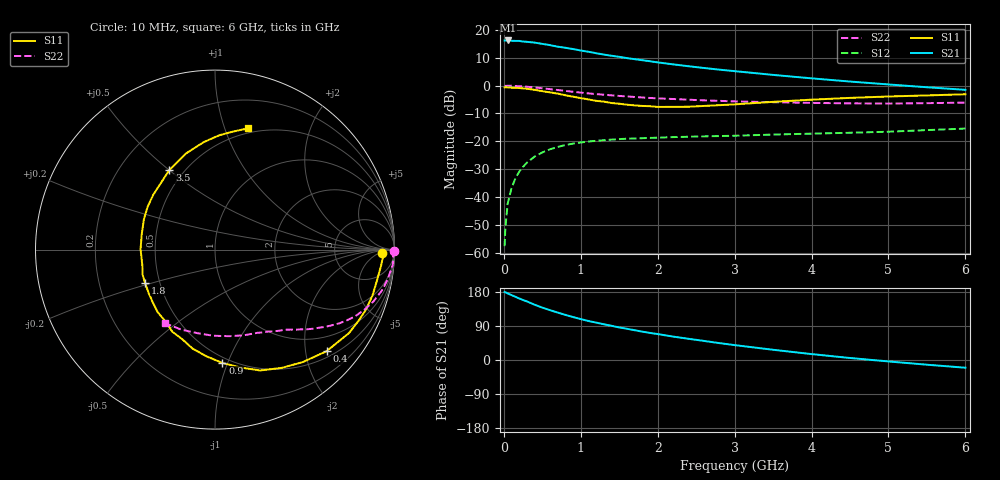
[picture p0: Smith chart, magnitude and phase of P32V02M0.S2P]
! SIEMENS Small Signal Semiconductors
! BFP181
! Si NPN RF Bipolar Junction Transistor in SOT143
! VCE = 2 V  IC = 2 mA
! Common Emitter S-Parameters:  March  1996
# GHz  S  MA  R  50
!  f  S11  S21  S12  S22
! GHz  MAG  ANG  MAG  ANG  MAG  ANG  MAG  ANG
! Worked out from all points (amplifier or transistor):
!   36 points, 10 MHz to 6 GHz, reference 50 ohm
!   highest |S21| = 16.2 dB at 50 MHz (marker M1)
!   |S21| within 3 dB of that: start of sweep to 881 MHz
!   unconditionally stable (mu >= 1): 2.395 GHz to end of sweep
!   at 250 MHz: K = 0.13, MSG = 22.5 dB, |S12| = -29.2 dB
!   at 1.4 GHz: K = 0.66, MSG = 15.1 dB, |S12| = -19.4 dB
!   at 6 GHz: K = 1.15, MAG = 4.6 dB, |S12| = -15.4 dB
!   lowest NFmin = 1.35 dB at 450 MHz
!   S11 on the Smith chart (normalised r, x): 10 MHz: 25, -8; 400 MHz: 0.63, -2.44; 900 MHz: 0.45, -0.96; 1.8 GHz: 0.41, -0.19; 3.5 GHz: 0.42, +0.50; 6 GHz: 0.45, +1.20
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0.01  0.9302 -1.3  6.469 179.4  0.0013 80.8  0.9969 -0.4
0.02  0.9375 -2.1  6.471 178.8  0.0028 89.9  0.9896 -0.9
0.05  0.9298 -5.5  6.487 175.6  0.0076 88.5  0.9938 -2.5
0.1  0.9185 -10.9  6.404 171.3  0.0144 82.8  0.9939 -4.9
0.2  0.905 -21.8  6.361 162.4  0.0284 76.6  0.9768 -9.6
0.3  0.8797 -31.9  6.126 154.6  0.0411 71.0  0.9553 -14.1
0.4  0.8408 -42.3  5.937 145.8  0.0531 65.2  0.9283 -18.2
0.5  0.7952 -52.0  5.629 138.2  0.0629 59.5  0.8962 -22.0
0.6  0.7561 -60.7  5.346 131.5  0.0717 54.7  0.8653 -25.4
0.7  0.719 -69.5  5.017 125.1  0.079 50.8  0.8337 -28.2
0.8  0.671 -78.0  4.796 119.0  0.0856 46.9  0.8049 -30.7
0.9  0.6326 -86.3  4.546 113.3  0.0908 43.5  0.775 -33.0
1.1  0.5653 -102.8  4.067 102.9  0.0988 37.9  0.725 -36.9
1.3  0.5156 -117.5  3.618 94.3  0.1046 33.0  0.686 -40.2
1.5  0.4727 -132.5  3.292 85.9  0.1093 29.9  0.6524 -42.9
1.8  0.4313 -154.8  2.864 74.8  0.1134 26.2  0.6123 -46.7
2.2  0.4148 179.6  2.412 61.8  0.1187 22.1  0.5748 -51.9
2.8  0.4453 147.3  1.938 44.6  0.124 18.6  0.5325 -60.1
3.5  0.5109 119.9  1.559 27.0  0.1319 15.8  0.5041 -71.2
4.5  0.6021 96.0  1.184 5.3  0.1422 12.6  0.4801 -91.1
5.5  0.6666 81.0  0.935 -12.4  0.1587 11.1  0.4838 -112.7
6  0.6996 74.8  0.84 -20.4  0.1691 9.1  0.4954 -123.9
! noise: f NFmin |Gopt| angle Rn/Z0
0.45  1.35  0.6  17  0.4
0.9  1.45  0.5  36  0.4
1.8  1.8  0.31  80  0.37
